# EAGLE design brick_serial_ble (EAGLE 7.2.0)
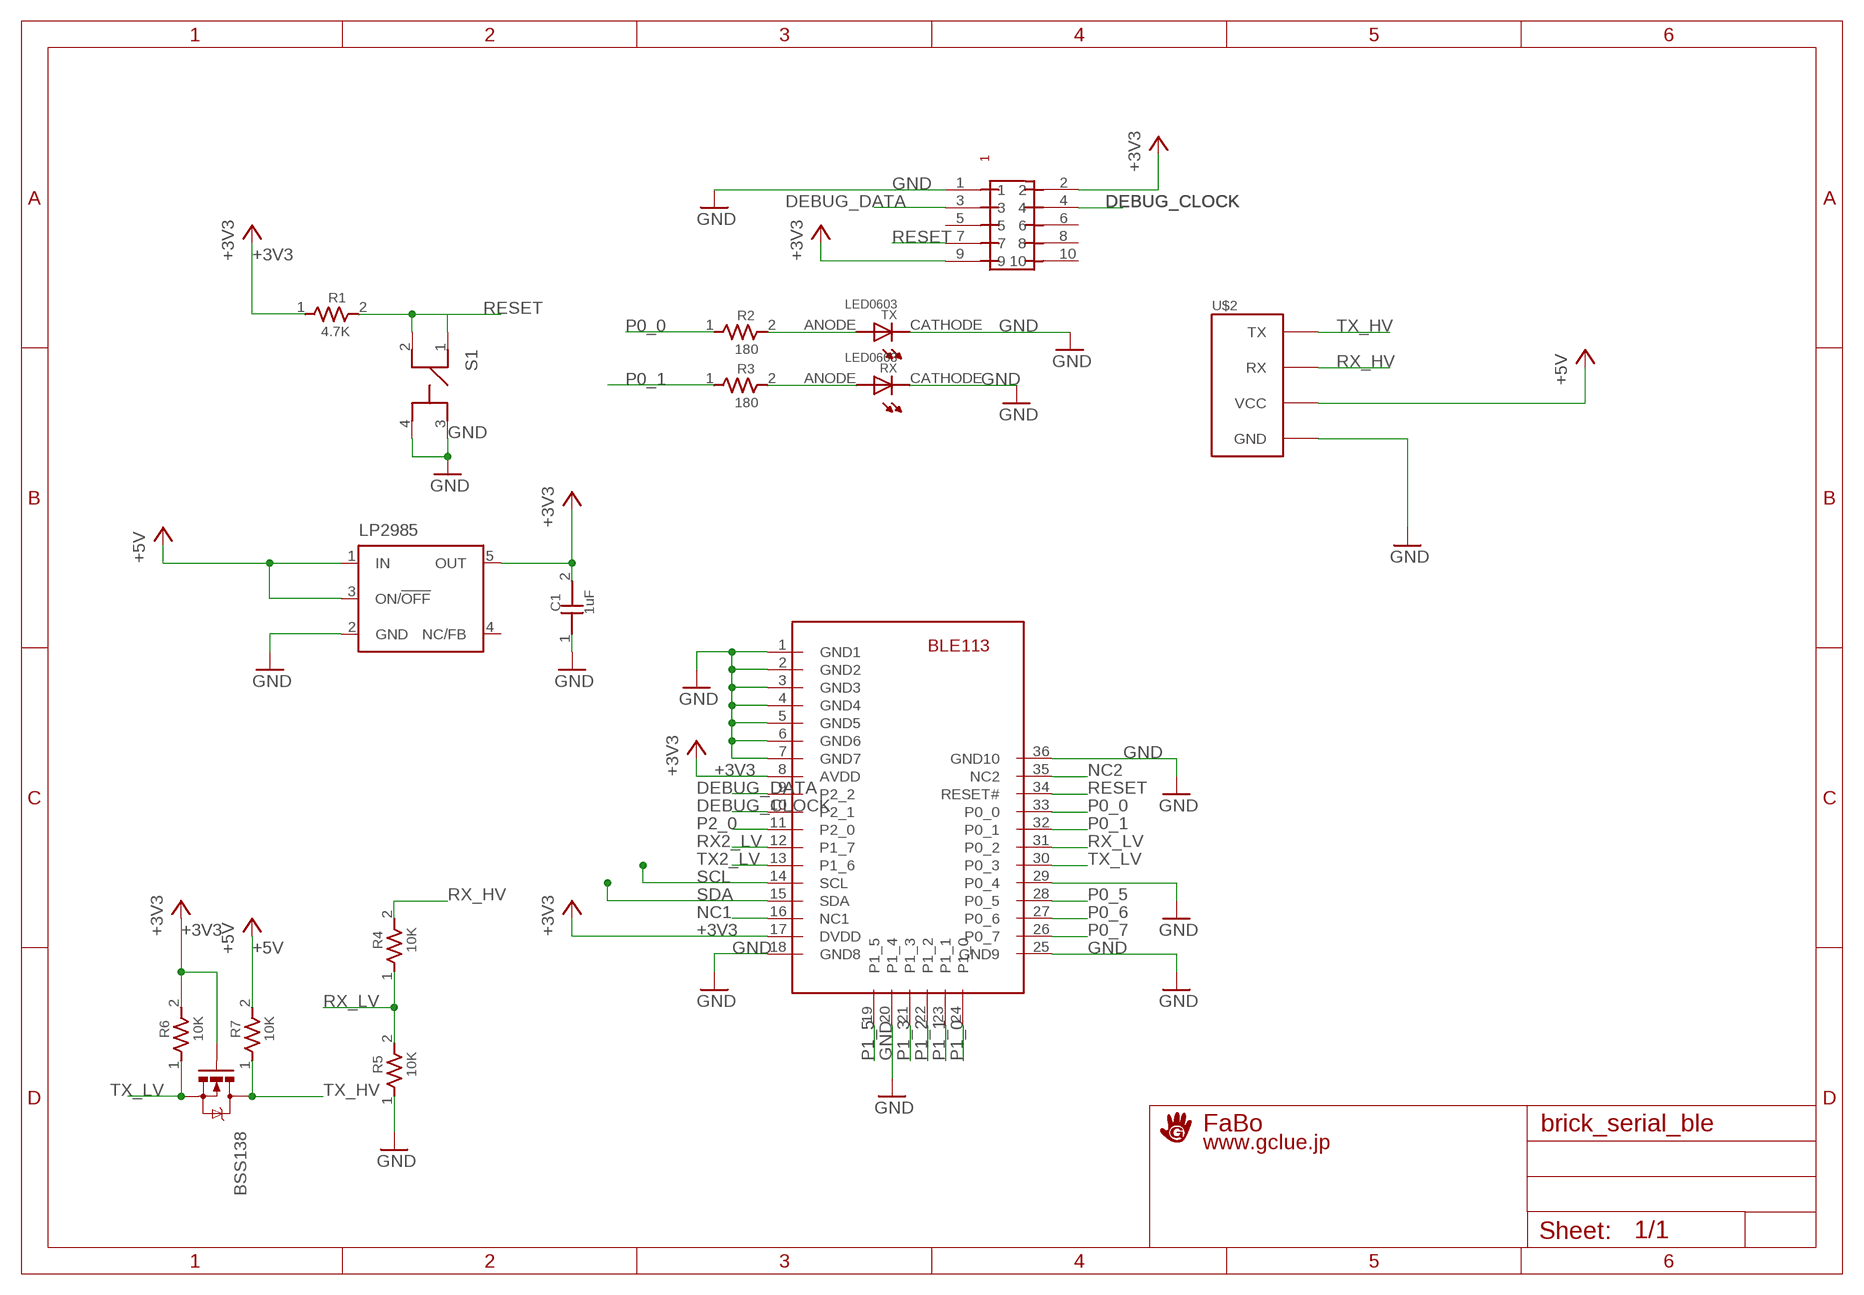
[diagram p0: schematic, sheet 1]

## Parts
BSS138  MOSFET-NCHANNELSMD  [SOT23-3]
C1  1uF  CAPACITOR0603  [0603]
LP2985  LP2985-XXDBVR33  [SOT23-DBV]
R1  4.7K  RESISTOR0603  [0603]
R2  180  RESISTOR0603  [0603]
R3  180  RESISTOR0603  [0603]
R4  10K  RESISTOR0603  [0603]
R5  10K  RESISTOR0603  [0603]
R6  10K  RESISTOR0603  [0603]
R7  10K  RESISTOR0603  [0603]
RX  LED0603  [0603]
S1  SWITCH-LS6J2M-T  [SWITCH-LS6J2M-T]
TX  LED0603  [0603]
U$1  PIN-HEADER-SMT(1.27MM)2X5  [PIN-HEADER-SMT(1.27MM)2X5]
U$2  BRICK_SERIAL  [BRICK_SERIAL]
U$3  LOGO_GCLUE-M  [LOGO_GCLUE_M]
U$6  BLUEGIGA-BLE113  [BLUEGIGA-BLE113]

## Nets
+3V3: BSS138.1(G) C1.2 LP2985.5(OUT) R1.1 R6.2 U$1.2 U$1.9 U$6.8(AVDD) U$6.17(DVDD)
+5V: LP2985.1(IN) LP2985.3(ON/!OFF) R7.2 U$2.VCC
DEBUG_CLOCK: U$1.4 U$6.10(P2_1)
DEBUG_DATA: U$1.3 U$6.9(P2_2)
GND: C1.1 LP2985.2(GND) R5.1 RX.CATHODE S1.3 S1.4 TX.CATHODE U$1.1 U$2.GND U$6.1(GND1) U$6.2(GND2) U$6.3(GND3) U$6.4(GND4) U$6.5(GND5) U$6.6(GND6) U$6.7(GND7) U$6.18(GND8) U$6.20(P1_4) U$6.25(GND9) U$6.29(P0_4) U$6.36(GND10)
N$1: R2.2 TX.ANODE
N$2: R3.2 RX.ANODE
NC1: U$6.16(NC1)
NC2: U$6.35(NC2)
P0_0: R2.1 U$6.33(P0_0)
P0_1: R3.1 U$6.32(P0_1)
P0_5: U$6.28(P0_5)
P0_6: U$6.27(P0_6)
P0_7: U$6.26(P0_7)
P1_0: U$6.24(P1_0)
P1_1: U$6.23(P1_1)
P1_2: U$6.22(P1_2)
P1_3: U$6.21(P1_3)
P1_5: U$6.19(P1_5)
P2_0: U$6.11(P2_0)
RESET: R1.2 S1.1 S1.2 U$1.7 U$6.34(RESET#)
RX2_LV: U$6.12(P1_7)
RX_HV: R4.2 U$2.RX
RX_LV: R4.1 R5.2 U$6.31(P0_2)
SCL: U$6.14(SCL)
SDA: U$6.15(SDA)
TX2_LV: U$6.13(P1_6)
TX_HV: BSS138.3(D) R7.1 U$2.TX
TX_LV: BSS138.2(S) R6.1 U$6.30(P0_3)
Unconnected: LP2985.4(NC/FB) U$1.5 U$1.6 U$1.8 U$1.10

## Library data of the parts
BSS138 = SparkFun:MOSFET-NCHANNEL
C1 = GClue-Capacitor:CAPACITOR
LP2985 = SmartPrj:LP2985-XXDBVR: ULTRALOW-POWER 50-mA LOW-DROPOUT LINEAR REGULATORS 50-mA Low-Dropout Regulator Source: http://focus.ti.com/lit/ds/symlink/tps77001.pdf
R1-R7 = GClue-Resistors:RESISTOR
RX TX = GClue-LED:LED
S1 = gclue:SWITCH-LS6J2M-T: Switch Tact SMD(LS6J2M-T)
U$1 = gclue:PIN-HEADER-SMT(1.27MM)2X5: PIN-HEADER-SMT (1.27MM) 2x5
U$2 = gclue:BRICK_SERIAL: FaBo Brick 4pin(SERIAL)
U$3 = gclue:LOGO_GCLUE
U$6 = gclueBT:BLUEGIGA-BLE113: Bluegiga BLE113 Bluetooth Bluetooth 4.0 low energy radio Radio Transmit power: +0 dBm Receiver sensitivity: -93 dBm Typical line-of-sight range: 30 - 100 meters Current Consumption TX peak current: 18.2 mA, 14.3 ma (with DC/DC) RX peak current: 17.9 mA Power mode 1: 270 uA Power mode 2: 1 uA Power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

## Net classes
0 default: width 0.254 mm, clearance 0.254 mm
2 GND: width 0.254 mm, drill 0.254 mm, clearance 0.254 mm
3 usbvcc: width 0.508 mm, drill 0.61 mm, clearance 0.254 mm

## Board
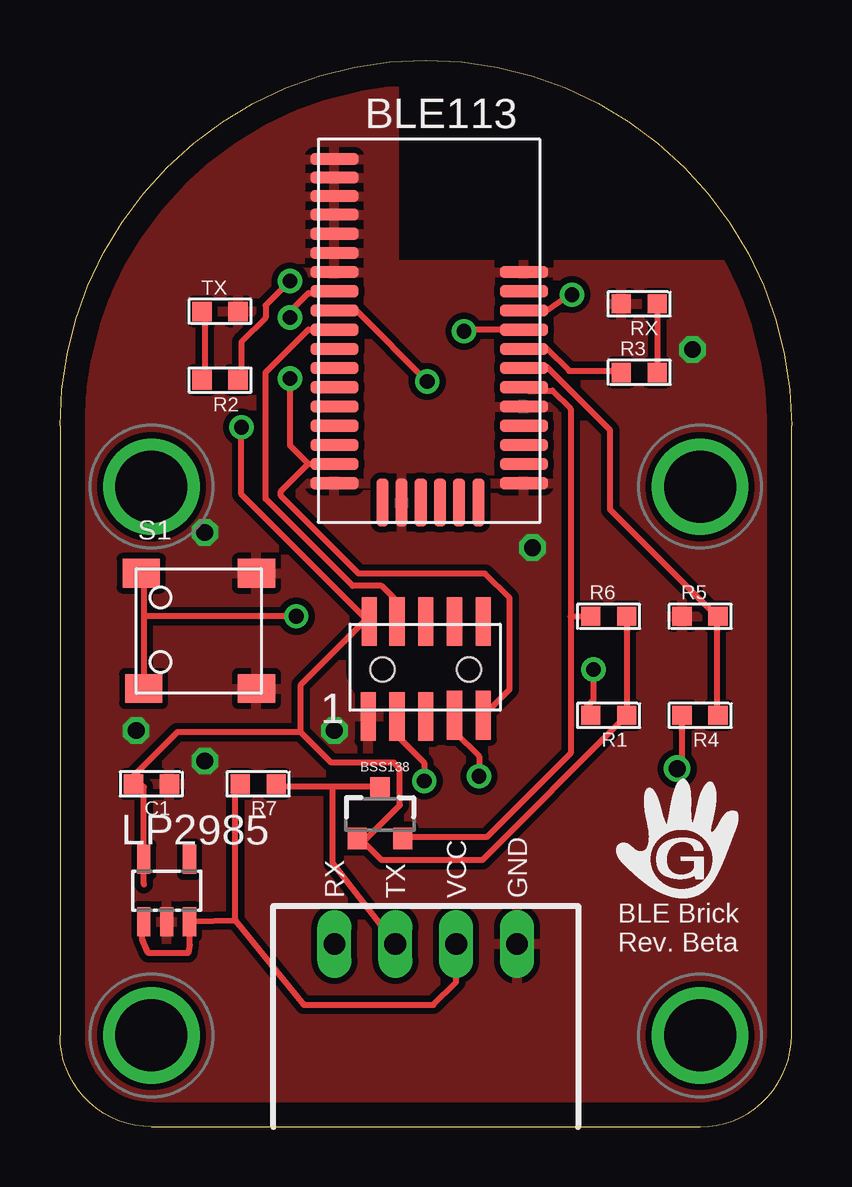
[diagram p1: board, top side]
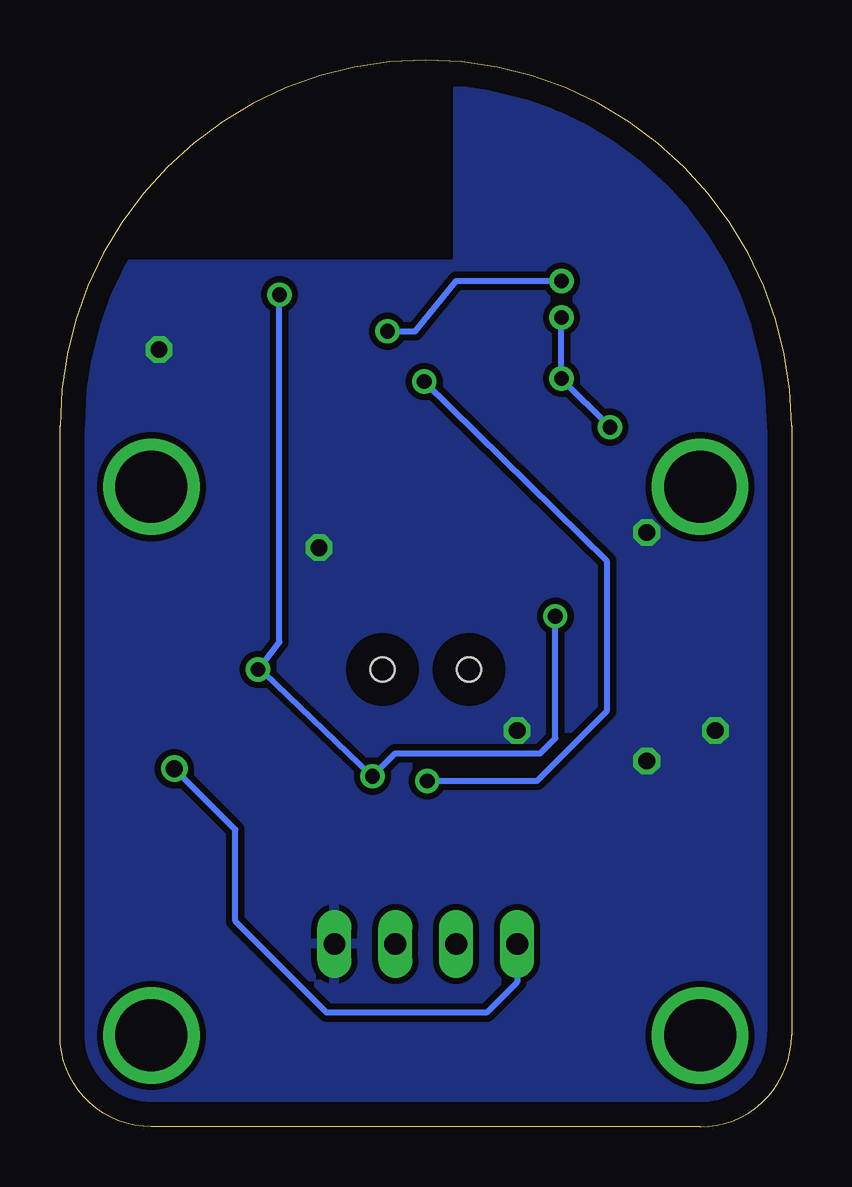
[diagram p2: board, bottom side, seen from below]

Size 30.48 x 44.45 mm. Coordinates in mm from the lower left corner, seen from the top.
Copper layers (1*16): Top 0.035mm / dielectric 1.5mm / Bottom 0.035mm
Design rules "default": minimum track width 10mil, minimum drill 24mil, track to track 8mil, track to pad 8mil, pad to pad 8mil, via to via 8mil, smd to smd 8mil, copper to edge 40mil, drill to drill 8mil, minimum pad ring 10mil, minimum via ring 8mil, stop-mask expansion 4mil, vias tented up to drill 0mil, thermal gap 10mil
tKeepout: area 14.2,35.9 to 32.2,45.9
bKeepout: area 14.2,35.9 to 32.2,45.9

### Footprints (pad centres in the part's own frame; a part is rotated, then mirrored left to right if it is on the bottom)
SOT23-3 = smd 0.8 x 0.9: 1 -0.95,-1; 2 0.95,-1; 3 0,1.1
0603 = smd 0.8 x 0.8: 1 -0.75,0; 2 0.75,0
SOT23-DBV = smd 0.55 x 1.2: 1 -0.95,-1.3; 2 0,-1.3; 3 0.95,-1.3; 4 0.95,1.3; 5 -0.95,1.3
0603' = smd 0.8 x 0.8: ANODE -0.75,0; CATHODE 0.75,0
SWITCH-LS6J2M-T = smd 1.55 x 1.2: 1 -2.4,2.4; 2 -2.3,-2.4; 3 2.4,2.4; 4 2.4,-2.4
PIN-HEADER-SMT(1.27MM)2X5 = smd 0.635 x 2.032: 1 -2.4,-1.95; 2 -2.35,2; 3 -1.2,-1.95; 4 -1.2,2; 5 0,-1.95; 6 0,2; 7 1.2,-1.9; 8 1.2,2; 9 2.4,-1.9; 10 2.4,2 | hole 1: 1.8,0; -1.8,0
BRICK_SERIAL = drill 0.9 long: GND 3.81,-11.43; RX -3.81,-11.43; TX -1.27,-11.43; VCC 1.27,-11.43 | drill 3 pad 3.81: P$5 -11.43,7.62; P$6 11.43,7.62; P$7 -11.43,-15.24; P$8 11.43,-15.24
BLUEGIGA-BLE113 = smd 2 x 0.5: 1 -3.81,6.35; 2 -3.81,5.58; 3 -3.81,4.81; 4 -3.81,4.04; 5 -3.81,3.24; 6 -3.81,2.44; 7 -3.81,1.64; 8 -3.81,0.84; 9 -3.81,0.04; 10 -3.81,-0.76; 11 -3.81,-1.56; 12 -3.81,-2.36; 13 -3.81,-3.16; 14 -3.81,-3.96; 15 -3.81,-4.76; 16 -3.81,-5.56; 17 -3.81,-6.36; 18 -3.81,-7.16; 25 4.09,-7.16; 26 4.09,-6.36; 27 4.09,-5.56; 28 4.09,-4.76; 29 4.09,-3.96; 30 4.09,-3.16; 31 4.09,-2.36; 32 4.09,-1.56; 33 4.09,-0.76; 34 4.09,0.04; 35 4.09,0.84; 36 4.09,1.64 | smd 0.5 x 2: 19 -1.81,-7.96; 20 -1.01,-7.96; 21 -0.21,-7.96; 22 0.59,-7.96; 23 1.39,-7.96; 24 2.19,-7.96

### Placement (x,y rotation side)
BSS138  13.34,13.02 0 top
C1  3.81,14.29 180 top
LP2985  4.45,9.84 0 top
R1  22.86,17.14 180 top
R2  6.67,31.12 180 top
R3  24.13,31.43 0 top
R4  26.67,17.14 180 top
R5  26.67,21.27 0 top
R6  22.86,21.27 0 top
R7  8.26,14.29 180 top
RX  LED0603  [0603']  24.13,34.29 180 top
S1  5.79,20.66 0 top
TX  LED0603  [0603']  6.67,33.97 0 top
U$1  15.24,19.05 0 top
U$2  15.24,19.05 0 top
U$3  25.72,12.06 0 top
U$6  15.24,33.97 0 top

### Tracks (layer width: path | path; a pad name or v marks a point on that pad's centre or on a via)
+3V3  (via drill 0.61)
  Top 0.254: 10.35,27.62 11.37,27.62 U$6.17 | 10.35,27.62 9.21,26.48 9.21,26.29 12.45,23.05 17.72,23.05 18.73,22.03 18.73,18.22 17.72,17.21 U$1.9 | v9.59,33.72 9.59,33.97 10.35,34.73 11.37,34.73 U$6.8 | v9.59,31.18 9.59,28.38 10.35,27.62 | LP2985.5 3.49,10.1 3.49,14.16 C1.2 2.86,14.41 4.89,16.45 10.03,16.45 | 12.64,11.87 13.4,11.11 17.59,11.11 23.43,16.95 R1.1 R6.2 | 10.03,16.45 10.03,18.41 12.64,21.02 U$1.2 12.64,21.27 7.56,26.35 v7.56,29.15 | 10.03,16.45 11.3,15.18 13.91,15.18 14.16,14.92 14.16,13.4 12.64,11.87 | 12.64,11.87 BSS138.1
  Bottom 0.254: v9.59,33.72 v9.59,31.18 v7.56,29.15
+5V
  Top 0.254: 7.3,8.6 7.3,14.16 R7.2 | 7.3,8.6 5.53,8.57 LP2985.3 5.4,7.62 5.33,7.24 3.68,7.24 3.43,7.81 3.43,8.32 LP2985.1 | U$2.VCC 16.51,6.03 15.56,5.08 10.16,5.08 7.3,8.6
DEBUG_CLOCK
  Top 0.254: U$6.10 11.37,33.21 10.35,33.21 8.57,31.43 8.57,26.16 12.19,22.54 13.4,22.54 13.91,22.03 13.91,21.27 U$1.4
DEBUG_DATA  (via drill 0.61)
  Top 0.254: v15.3,31.05 12.38,33.97 11.62,33.97 U$6.9 | v15.18,14.41 15.18,15.18 14.16,16.19 14.16,16.95 U$1.3
  Bottom 0.254: v15.3,31.05 7.68,23.56 7.68,17.34 10.6,14.41 v15.18,14.41
GND  (via drill 0.7)
  other vias: 19.69,24.13 6.03,24.77 3.18,16.51 26.35,32.38 11.43,16.51 6.03,15.24
  pour Top: -0.55,-0.82 -0.55,46.13 13.9,46.13 13.9,35.91 30.45,35.91 30.45,-0.82
  pour Bottom: -0.55,-0.82 -0.55,46.13 13.9,46.13 13.9,35.91 30.45,35.91 30.45,-0.82
N$1
  Top 0.254: R2.2 6.03,31.18 6.03,33.97 TX.ANODE
N$2
  Top 0.254: R3.2 24.89,31.18 24.89,33.97 RX.ANODE
P0_0  (via drill 0.61)
  Top 0.254: v9.59,35.24 8.57,34.23 8.57,33.72 7.56,32.7 7.56,31.18 R2.1 | U$6.33 16.89,33.21 v16.83,33.15
  Bottom 0.254: v9.59,35.24 13.97,35.24 15.69,33.15 v16.83,33.15
P0_1
  Top 0.254: R3.1 23.37,31.5 21.21,31.5 20.26,32.45 19.49,32.45 U$6.32
RESET  (via drill 0.61)
  Top 0.254: 3.49,21.27 3.49,23.05 S1.1 | 3.49,21.27 3.49,18.48 S1.2 | v22.23,19.05 22.23,17.78 21.91,17.46 21.91,17.15 R1.2 | v17.46,14.6 17.46,15.43 16.45,16.45 16.45,16.95 U$1.7 | v21.34,34.67 21.34,34.73 20.26,33.97 19.49,33.97 U$6.34 | v9.84,21.27 3.49,21.27
  Bottom 0.254: v21.34,34.67 21.34,20.19 v22.23,19.05 21.97,18.92 v17.46,14.6 16.51,15.56 10.48,15.56 9.84,16.19 v9.84,21.27
RX_HV  (via drill 0.7)
  Top 0.254: v25.72,14.92 25.92,15.13 R4.2
  Bottom 0.254: v25.72,14.92 23.18,12.38 23.18,8.57 19.37,4.76 12.7,4.76 11.43,6.03 U$2.RX
RX_LV
  Top 0.254: 27.37,21.27 27.37,17.21 R4.1 | 27.37,21.27 22.92,25.72 22.92,29.02 20.26,31.69 19.49,31.69 U$6.31 | 27.37,21.27 R5.2
TX_HV
  Top 0.254: 11.37,14.16 13.14,14.16 BSS138.3 | 11.37,14.16 9.08,14.16 R7.1 | 11.37,14.16 11.37,10.99 U$2.TX
TX_LV
  Top 0.254: 21.27,21.27 21.27,29.91 20.51,30.67 19.49,30.67 U$6.30 | 21.27,21.27 21.27,15.56 17.78,12.07 14.29,12.07 BSS138.2 | 21.27,21.27 R6.1

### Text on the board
tPlace: BLE Brick / Rev. Beta

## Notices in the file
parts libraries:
SparkFun: Licensing: CC v3.0 Share-Alike You are welcome to use this library for commercial purposes.
